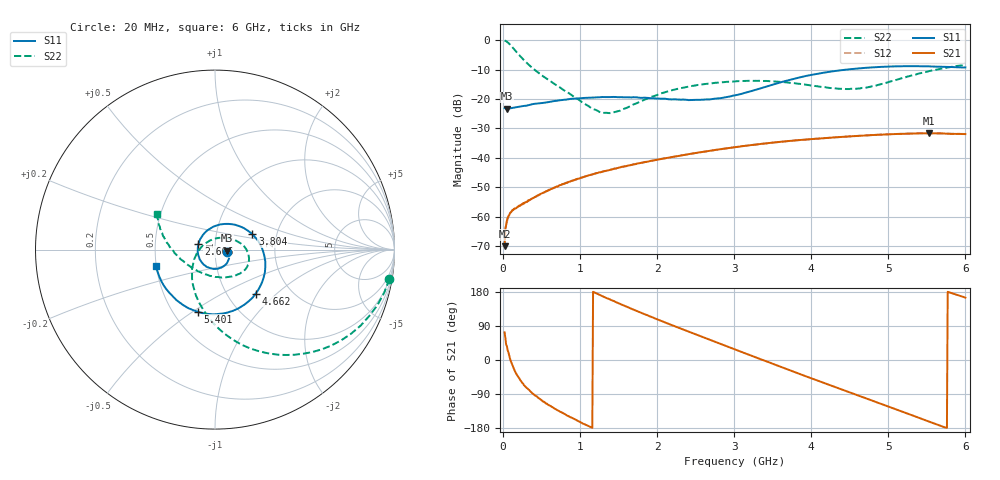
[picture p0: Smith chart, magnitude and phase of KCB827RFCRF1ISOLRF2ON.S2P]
!Agilent Technologies,E5071B,JP1KK00126,A.08.11
!Date: Tue May 06 07:34:24 2014
!Data & Calibration Information:
!Freq	S11:SOLT2(ON)	S21:SOLT2(ON)	S12:SOLT2(ON)	S22:SOLT2(ON)
# Hz S dB R 50
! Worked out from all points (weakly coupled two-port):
!   600 points, 20 MHz to 6 GHz, reference 50 ohm
!   highest |S21| = -31.67 dB at 5.531 GHz (marker M1); lowest = -70.0 dB at 20 MHz (marker M2)
!   lowest |S11| = -23.3 dB at 49.95 MHz (marker M3), VSWR 1.15, Z = 57.3 - j0.706 ohm
!   |S11| at or under -10 dB: start of sweep to 4.469 GHz
!   |S22| runs from -24.8 to -0.1 dB; largest |S21 - S12| = 0.00022
!   S11 on the Smith chart (normalised r, x): 20 MHz: 1.15, -0.04; 2.606 GHz: 0.83, +0.05; 3.804 GHz: 1.50, +0.27; 4.662 GHz: 1.35, -0.74; 5.401 GHz: 0.66, -0.53; 6 GHz: 0.50, -0.11
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2e7  -23.06 -12.7  -70.03 73.0  -69.11 63.4  -0.13 -9.6
4.994992e7  -23.30 -5.1  -61.30 36.3  -61.91 33.6  -0.58 -23.3
7.989983e7  -23.22 -4.0  -59.48 11.4  -59.34 10.4  -1.25 -35.7
1.397997e8  -22.95 -4.3  -57.40 -23.1  -57.56 -23.2  -2.99 -56.0
2.196661e8  -22.54 -6.2  -56.29 -51.8  -56.36 -51.8  -5.39 -75.7
3.194992e8  -22.18 -11.7  -54.82 -75.5  -54.58 -74.8  -8.04 -93.2
5.690818e8  -21.16 -25.5  -51.33 -115.3  -51.31 -116.0  -13.16 -125.0
1.018331e9  -19.70 -58.4  -46.74 -165.5  -46.74 -165.6  -21.00 -177.4
1.25793e9  -19.44 -78.2  -44.92 171.3  -44.91 170.9  -24.48 138.1
1.387713e9  -19.36 -88.7  -44.15 160.1  -44.13 159.7  -24.82 108.3
2.016661e9  -19.90 -141.7  -40.55 106.3  -40.58 105.9  -18.44 26.7
2.605676e9  -20.24 161.0  -37.94 59.3  -37.95 59.5  -14.99 -1.7
3.014992e9  -18.75 111.0  -36.37 27.5  -36.38 27.4  -14.03 -18.1
3.444274e9  -15.57 59.0  -34.99 -5.5  -35.00 -5.8  -13.94 -34.2
3.803673e9  -12.96 22.5  -34.06 -33.5  -34.07 -33.6  -14.73 -51.5
4.013322e9  -11.76 3.8  -33.65 -49.3  -33.63 -49.4  -15.47 -65.2
4.342771e9  -10.38 -23.0  -33.01 -73.8  -33.01 -74.1  -16.49 -93.4
4.662237e9  -9.53 -47.2  -32.47 -97.6  -32.47 -97.8  -16.24 -128.1
5.011653e9  -9.00 -73.3  -32.01 -123.7  -32.01 -124.0  -14.18 -163.1
5.401002e9  -8.89 -105.4  -31.67 -153.0  -31.66 -153.1  -11.34 171.9
5.530785e9  -8.94 -117.1  -31.67 -162.7  -31.65 -162.9  -10.52 165.6
6e9  -9.29 -164.2  -31.95 164.5  -31.93 164.5  -8.42 148.3
